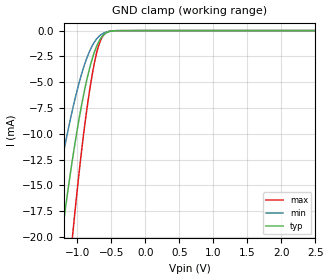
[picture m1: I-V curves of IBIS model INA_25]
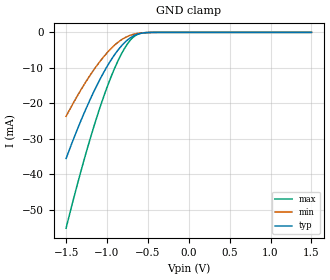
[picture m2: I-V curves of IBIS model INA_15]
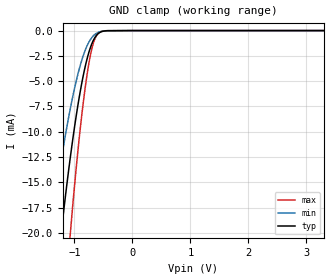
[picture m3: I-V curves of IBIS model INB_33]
| TEXAS INSTRUMENTS INCORPORATED
| Standard Linear and Logic Group / High Volume Linear
| IBIS Model of TCA9509
| Level Translating I2C/SMBUS Bus Repeater
| This file contains package information for the following:
|  SOT 8-pin (DCT) package as [Component] TCA9509_DCT
| This device can be powered at the following Vccs:
|  3.3 volt Vcc
|  2.5 volt Vcc
|  1.8 volt Vcc
|  1.5 volt Vcc
|  1.2 volt Vcc
| This file provides unique models under the [Model Selector] for each Vcc.
| For operation at a specific Vcc, select the appropriate model after each
| [Model Selector] keyword.
[IBIS Ver]   3.2
[Comment char]  |_char
[File Name]   tca9509.ibs
[File Rev]   0 | A0
[Date]   January 24, 2011
[Source]   Data created from TI-SPICE simulations at TI-SLL/HVL.
   The following is an IBIS list for the TCA9509.
   Please contact sllibis@ti.com with questions and
   comments concerning SLL IBIS models.
[Notes]   Revision_History:
##notes##|
[Disclaimer]
| This model is designed as an aid for customers of Texas Instruments.
| TI and its licensors and suppliers make no warranties, either expressed
| or implied, with respect to this  model, including the warranties of
| merchantability or fitness for a particular purpose. The model is
| provided solely on an "as is" basis. The entire risk as to its quality
| and performance is with the customer.
[Copyright]
| (C) Copyright 2011 Texas Instruments Incorporated. All rights reserved.
| Component TCA9509_RVH 8-PIN QFN
[Component]   TCA9509_RVH
[Manufacturer]   Texas Instruments, Inc.
[Package]
|   typ   min   max
R_pkg   5.475e-02   4.963e-02   6.255e-02
L_pkg   5.888e-10   5.356e-10   6.638e-10
C_pkg   7.783e-14   7.051e-14   8.266e-14
[Pin]   signal_name   model_name   R_pin   L_pin   C_pin
1   VCCA   POWER   5.498e-02   6.065e-10   7.919e-14
2   SCLA   INA   5.014e-02   5.479e-10   7.135e-14
3   SDAA   OUTA   6.255e-02   6.638e-10   8.231e-14
4   GND   GND   5.343e-02   5.764e-10   8.266e-14
5   EN   ENA   6.071e-02   5.399e-10   7.983e-14
6   SDAB   INB   4.963e-02   5.356e-10   7.051e-14
7   SCLB   OUTB   5.648e-02   5.967e-10   7.669e-14
8   VCCB   POWER   5.010e-02   5.437e-10   8.008e-14
| Model INA
[Model Selector]   INA
INA_33   3.3 volt Vcc
INA_25   2.5 volt Vcc
INA_18   1.8 volt Vcc
INA_15   1.5 volt Vcc
INA_12   1.2 volt Vcc
| Model INB
[Model Selector]   INB
INB_33   3.3 volt Vcc
INB_25   2.5 volt Vcc
INB_18   1.8 volt Vcc
INB_15   1.5 volt Vcc
INB_12   1.2 volt Vcc
| Model ENA
[Model Selector]   ENA
ENA_33   3.3 volt Vcc
ENA_25   2.5 volt Vcc
ENA_18   1.8 volt Vcc
ENA_15   1.5 volt Vcc
ENA_12   1.2 volt Vcc
| Model OUTA
[Model Selector]   OUTA
OUTA_33   3.3 volt Vcc
OUTA_25   2.5 volt Vcc
OUTA_18   1.8 volt Vcc
OUTA_15   1.5 volt Vcc
OUTA_12   1.2 volt Vcc
| Model OUTB
[Model Selector]   OUTB
OUTB_33   3.3 volt Vcc
OUTB_25   2.5 volt Vcc
OUTB_18   1.8 volt Vcc
OUTB_15   1.5 volt Vcc
OUTB_12   1.2 volt Vcc
| Models and submodels in the file (25): INA_33 (Input), INA_25 (Input), INA_18 (Input), INA_15 (Input), INA_12 (Input), INB_33 (Input), INB_25 (Input), INB_18 (Input), INB_15 (Input), INB_12 (Input), ENA_33 (Input), ENA_25 (Input), ENA_18 (Input), ENA_15 (Input), ENA_12 (Input), OUTA_33 (Open_drain), OUTA_25 (Open_drain), OUTA_18 (Open_drain), OUTA_15 (Open_drain), OUTA_12 (Open_drain), OUTB_33 (Open_drain), OUTB_25 (Open_drain), OUTB_18 (Open_drain), OUTB_15 (Open_drain), OUTB_12 (Open_drain)
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[Model]   INA_25
Model_type  Input
Vinl=0.15
Vinh=1.75
| variable   typ   min   max
C_comp   1.62pF   1.22pF   1.89pF
[Temperature Range]   40   100   -40
| Ambient temperature   25   85   -40
[Voltage range]   2.5   2.3   2.7
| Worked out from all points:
|   GND clamp passes 1 mA (typ) near -0.68 V on its own axis
[GND Clamp]
| INA_25
|   Voltage   I(typ)   I(min)   I(max)
-2.5V     -109.9mA   -78.03mA   -160.4mA
-1.405V   -29.79mA   -19.62mA   -46.56mA
-1.21V    -19.12mA   -12.2mA    -30.31mA
-1.075V   -12.75mA   -7.861mA   -20.42mA
-1.055V   -11.89mA   -7.281mA   -19.07mA
-920mV    -6.722mA   -3.883mA   -10.84mA
-805mV    -3.354mA   -1.825mA   -5.303mA
-710mV    -1.465mA   -779.9uA   -2.066mA
-625mV    -513.9uA   -292.4uA   -560.9uA
-545mV    -136.8uA   -94.94uA   -106.9uA
-430mV    -13.52uA   -13.5uA    -5.631uA
2.5V      247.4pA    1.266nA    41.34pA
[Model]   INA_15
Model_type  Input
Vinl=0.15
Vinh=1.05
| variable   typ   min   max
C_comp   1.59pF   1.11pF   1.82pF
[Temperature Range]   40   100   -40
| Ambient temperature   25   85   -40
[Voltage range]   1.5   1.35   1.65
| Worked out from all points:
|   GND clamp passes 1 mA (typ) near -0.68 V on its own axis
[GND Clamp]
| INA_15
|   Voltage   I(typ)   I(min)   I(max)
-1.5V     -35.53mA   -23.65mA   -55.14mA
-1.375V   -28.05mA   -18.4mA    -43.93mA
-1.255V   -21.44mA   -13.8mA    -33.88mA
-1.14V    -15.7mA    -9.862mA   -25.02mA
-1.035V   -11.06mA   -6.72mA    -17.75mA
-935mV    -7.237mA   -4.213mA   -11.67mA
-840mV    -4.263mA   -2.36mA    -6.822mA
-750mV    -2.153mA   -1.149mA   -3.25mA
-670mV    -934.3uA   -505.3uA   -1.19mA
-595mV    -324.9uA   -196.1uA   -314.7uA
-480mV    -38.67uA   -33.04uA   -22.02uA
1.5V      175.6pA    965.7pA    24.92pA
[Model]   INB_33
Model_type  Input
Vinl=0.15
Vinh=2.31
| variable   typ   min   max
C_comp   1.60pF   1.24pF   1.83pF
[Temperature Range]   40   100   -40
| Ambient temperature   25   85   -40
[Voltage range]   3.3   3   3.6
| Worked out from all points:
|   GND clamp passes 1 mA (typ) near -0.68 V on its own axis
[GND Clamp]
| INB_33
|   Voltage   I(typ)   I(min)   I(max)
-3.3V     -179.4mA   -131.1mA   -253.4mA
-1.42V    -30.67mA   -20.24mA   -47.89mA
-1.4V     -29.5mA    -19.42mA   -46.12mA
-1.22V    -19.63mA   -12.55mA   -31.1mA
-1.07V    -12.54mA   -7.714mA   -20.08mA
-920mV    -6.722mA   -3.883mA   -10.84mA
-805mV    -3.354mA   -1.825mA   -5.303mA
-705mV    -1.39mA    -740.7uA   -1.939mA
-645mV    -679uA     -375.8uA   -797.3uA
-595mV    -324.9uA   -196.1uA   -314.7uA
-435mV    -15.07uA   -14.81uA   -6.498uA
3.3V      311.6pA    1.532nA    54.55pA
